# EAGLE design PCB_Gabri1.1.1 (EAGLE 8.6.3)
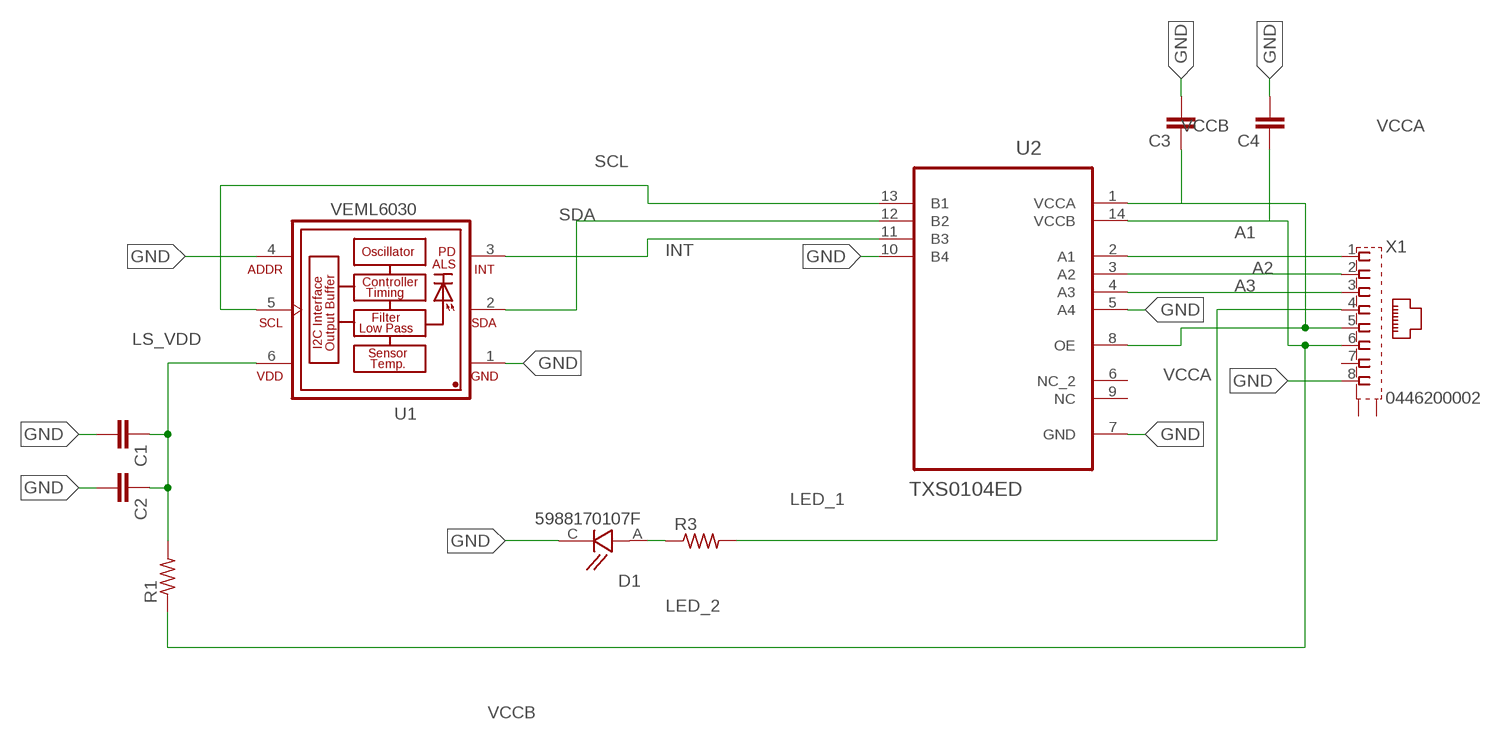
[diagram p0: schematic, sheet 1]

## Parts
C1  C-EU025-024X044  [C025-024X044]
C2  C-EU025-024X044  [C025-024X044]
C3  C-EU025-024X044  [C025-024X044]
C4  C-EU025-024X044  [C025-024X044]
D1  5988170107F  [LEDC2012X70N]
R1  R-US_R0805  [R0805]
R3  R-US_R0805  [R0805]
U1  VEML6030  [VISHAY_VEML6030_2X2X0.87]
U2  TXS0104ED  [SOIC127P600X175-14N]
X1  0446200002  [0446200002]

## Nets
A1: U2.2(A1) X1.1
A2: U2.3(A2) X1.2
A3: U2.4(A3) X1.3
GND: C1.2 C2.2 C3.2 C4.2 D1.C U1.1(GND) U1.4(ADDR) U2.5(A4) U2.7(GND) U2.10(B4) X1.8
INT: U1.3(INT) U2.11(B3)
LED_1: R3.2 X1.4
LED_2: D1.A R3.1
LS_VDD: C1.1 C2.1 R1.2 U1.6(VDD)
SCL: U1.5(SCL) U2.13(B1)
SDA: U1.2(SDA) U2.12(B2)
VCCA: C3.1 U2.1(VCCA) U2.8(OE) X1.5
VCCB: C4.1 R1.1 U2.14(VCCB) X1.6
Unconnected: U2.6(NC_2) U2.9(NC) X1.7 X1.S@1(S1) X1.S@2(S2)

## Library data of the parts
C1-C4 = resistor:C-EU: CAPACITOR, European symbol
D1 = 5988170107F:5988170107F: Standard LEDs - SMD Green Water Clr 40mcd 570nm; AVAILABILITY: Unavailable; DESCRIPTION: LED GREEN CLEAR 0805 SMD; MF: Dialight; MP: 5988170107F; PACKAGE: 0805 Dialight; PRICE: None
R1 R3 = resistor:R-US_: RESISTOR, American symbol
U1 = VEML6030:VEML6030: VEML6030 High Accuracy Ambient Light Sensor with I2C Interface: VEML6030 is a high accuracy ambient light digital 16-bit resolution sensor in a miniature transparent 2 mm x 2 mm package. It includes a high sensitive photodiode, a low noise amplifier, a 16-bit A/D converter and supports an easy to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; AVAILABILITY: Unavailable; DESCRIPTION: VEML6030 Series 2 x 2 x 0.85 mm 50 mW I2C High Accuracy Ambient Light Sensor; MF: Vishay; MP: VEML6030; PACKAGE: SMD-6 Vishay; PRICE: None
U2 = TXS0104ED:TXS0104ED: 4-BIT BIDIRECTIONAL VOLTAGE-LEVEL TRANSLATOR FOR OPEN-DRAIN AND PUSH-PULL APPLICATIONS; AVAILABILITY: Unavailable; DESCRIPTION: 4-Bit Bidirectional Voltage-Level Shifter for Open-Drain and Push-Pull Applications 14-SOIC -40 to 85; MF: Texas Instruments; MP: TXS0104ED; PACKAGE: SOIC-14 Texas Instruments; PRICE: None
X1 = 0446200002:0446200002: RJ-45 INVERTED MODULAR JACK ASSEMBLY WITH RJ-11 KEEPOUT FEATURE Source: Data sheet MOLEX 0446200002 BUCHSE, RJ45, GESCHIRMT Source: Farnell; AVAILABILITY: Unavailable; DESCRIPTION: Conn RJ-45 RCP 8 POS 2.04mm Solder RA Thru-Hole 8 Terminal 1 Port Tray Cat 3; MF: Molex, LLC; MP: 0446200002; PACKAGE: None; PRICE: None

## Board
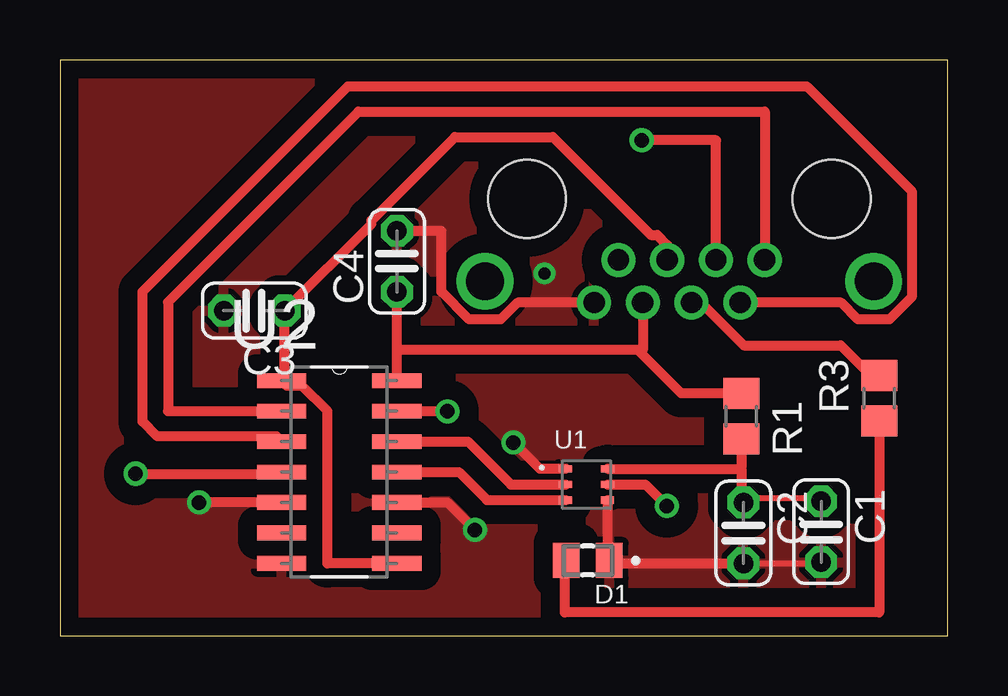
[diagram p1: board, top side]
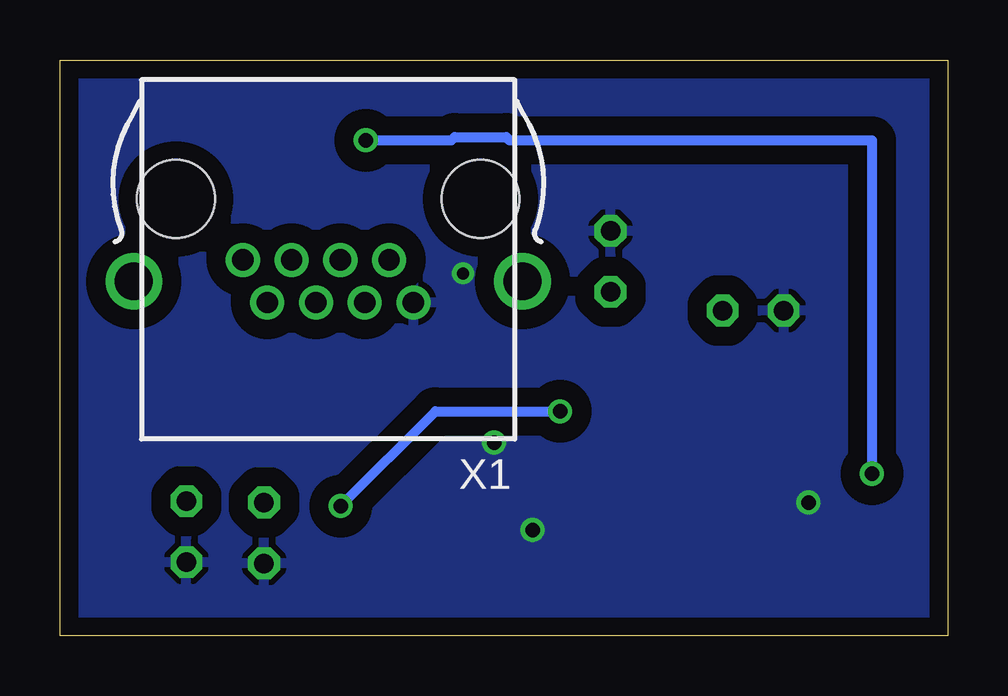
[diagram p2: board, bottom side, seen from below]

Size 37 x 24 mm. Coordinates in mm from the lower left corner, seen from the top.
Outline: 0,0 37,0 37,24 0,24 0,0
Copper layers (1*16): Top 0.035mm / dielectric 1.5mm / Bottom 0.035mm
Design rules "default *": minimum track width 10mil, minimum drill 0.5mm, track to track 0.8mm, track to pad 8mil, pad to pad 8mil, via to via 8mil, smd to smd 8mil, copper to edge 30mil, drill to drill 8mil, minimum pad ring 10mil, minimum via ring 8mil, stop-mask expansion 4mil, vias tented up to drill 0mil, thermal gap 10mil

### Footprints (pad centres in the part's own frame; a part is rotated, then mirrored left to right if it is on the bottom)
C025-024X044 = drill 0.813 octagon: 1 -1.27,0; 2 1.27,0
LEDC2012X70N = smd 1.1 x 1.45: A 0.9,0; C -0.9,0
R0805 = smd 1.3 x 1.5: 1 -0.95,0; 2 0.95,0
VISHAY_VEML6030_2X2X0.87 = smd 0.55 x 0.3: 1 -0.875,0.65; 2 -0.875,0; 3 -0.875,-0.65; 4 0.875,-0.65; 5 0.875,0; 6 0.875,0.65
SOIC127P600X175-14N = smd 2.057 x 0.61: 1 -4.801,7.62; 2 -4.801,6.35; 3 -4.801,5.08; 4 -4.801,3.81; 5 -4.801,2.54; 6 -4.801,1.27; 7 -4.801,0; 8 0,0; 9 0,1.27; 10 0,2.54; 11 0,3.81; 12 0,5.08; 13 0,6.35; 14 0,7.62
0446200002 = drill 0.889 pad 1.422: 1 3.556,2.54; 2 2.54,4.318; 3 1.524,2.54; 4 0.508,4.318; 5 -0.508,2.54; 6 -1.524,4.318; 7 -2.54,2.54; 8 -3.556,4.318 | drill 1.575 pad 2.286: S@1 -8.103,3.429; S@2 8.103,3.429 | hole 3.251: 6.35,0; -6.35,0

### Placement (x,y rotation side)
C1  31.73,4.33 270 top
C2  28.49,4.28 270 top
C3  8.1,13.55 180 top
C4  14.05,15.6 90 top
D1  22,3.13 180 top
R1  28.4,9.15 270 top
R3  34.15,9.9 90 top
U1  21.95,6.3 0 top
U2  14.04,3.01 0 top
X1  25.82,18.2 180 bottom

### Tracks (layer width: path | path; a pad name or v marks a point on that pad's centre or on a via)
A1
  Top 0.406: U2.2 4.5,9.36 4.5,13.9 12.45,21.85 29.38,21.85 X1.1
A2
  Top 0.406: U2.3 9.03,8.3 4.06,8.3 3.44,8.92 3.44,14.34 12.01,22.9 31.13,22.9 35.51,18.52 35.51,14.11 34.58,13.18 33.27,13.18 32.57,13.88 X1.2
A3  (via drill 0.6)
  Top 0.406: X1.3 27.34,20.65 v24.25,20.65 | v3.15,6.75 9.24,6.75 U2.4
  Bottom 0.406: v24.25,20.65 20.68,20.65 20.54,20.79 18.4,20.79 18.26,20.65 3.15,20.65 v3.15,6.75
GND  (via drill 0.5, 0.6)
  Top 0.254: C1.2 31.5,3.02 28.78,3.02 28.64,3.02 C2.2
  Top 0.406: 28.64,3.02 22.9,3.02 D1.C 22.83,3.13 U1.4 | U1.1 20,6.95 v18.9,8.05 | U2.10 16.15,5.55 v17.3,4.4 | X1.8 19.07,13.88 18.38,13.18 17.06,13.18 15.9,14.34 15.9,16.87 C4.2 | U2.5 v5.8,5.55
  other vias: 20.2,15.1
  pour Bottom: 0.25,23.8 0.25,0.25 36.85,0.25 36.85,23.8
  pour Top: 0.4,23.55 0.4,0.35 36.6,0.35 36.6,23.55
INT
  Top 0.406: U1.3 17.8,5.65 16.63,6.82 U2.11
LED_1
  Top 0.406: X1.4 26.72,13.88 28.51,12.1 32.55,12.1 33.8,10.85 R3.2
LED_2
  Top 0.406: R3.1 34.15,0.97 21.05,0.97 21.05,3.13 D1.A
LS_VDD
  Top 0.254: C1.1 31.5,5.73 28.78,5.73 28.59,5.61 C2.1
  Top 0.406: 28.4,6.95 28.4,5.61 28.59,5.61 | U1.6 28.4,6.95 | 28.4,6.95 28.4,7 R1.2
SCL  (via drill 0.6)
  Top 0.406: U1.5 24.4,6.3 v25.3,5.4 | v16.15,9.35 U2.13
  Bottom 0.406: v25.3,5.4 21.35,9.35 v16.15,9.35
SDA
  Top 0.406: U1.2 18.8,6.3 17.01,8.09 U2.12
VCCA
  Top 0.406: X1.5 25.31,16.29 24.9,16.7 24.63,16.7 20.54,20.79 16.46,20.79 12.98,17.31 12.98,17.16 C3.1 9.37,10.7 9.24,10.57 U2.1 9.45,10.42 10.09,10.42 11.15,9.36 11.15,3.01 U2.8
VCCB
  Top 0.406: U2.14 14.05,11.9 | 14.05,11.9 C4.1 | X1.6 24.3,11.9 24.1,11.9 | 24.1,11.9 14.05,11.9 | R1.1 25.9,10.1 24.1,11.9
